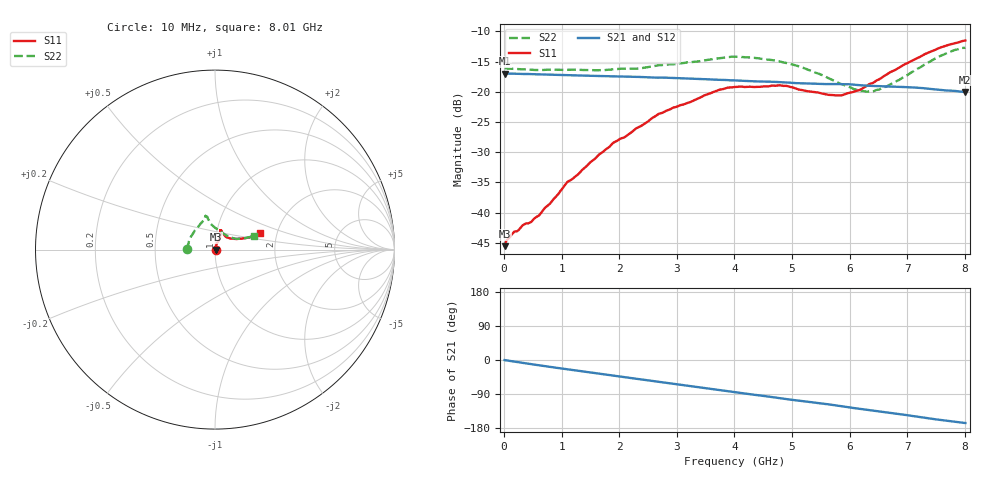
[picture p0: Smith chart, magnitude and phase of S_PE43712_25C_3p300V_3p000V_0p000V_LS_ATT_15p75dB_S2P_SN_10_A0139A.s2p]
! DEVICE ID: PE43712
! File Path: z:\PE43713\PE43713_CHAR_NOM_04292014\AMB\3p300\LS_ATT_15p75dB\PE43713_AMB_3p300V_3p000V_0p000V_LS_ATT_15p75dB_S2P_SN_10_A0139A.s2p
! Serial: 10
! Lot: A0139A
! Temp: 25C
! VDD: 3.300
! VSS: 0.000
! Control_Hi: 3.000
! Control_Lo: 0.000
! Attenuation Step: 15.75dB
! Port 1: RF1
! Port 2: RF2
! ThroughPath:1-2
! IDD: 0.0001475345
! ISS: -1.669e-007
#  Hz  S  RI  R  50
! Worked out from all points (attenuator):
!   801 points, 10 MHz to 8.01 GHz, reference 50 ohm
!   highest |S21| = -16.97 dB at 10 MHz (marker M1); lowest = -20.0 dB at 8 GHz (marker M2)
!   lowest |S11| = -45.6 dB at 10 MHz (marker M3), VSWR 1.01, Z = 50.5 + j0.0439 ohm
!   |S11| at or under -10 dB: start of sweep to end of sweep
!   |S22| runs from -20.0 to -12.7 dB; largest |S21 - S12| = 0.00053
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1e7  0.00525 0.000435  0.1418 -0.000698  0.1419 -0.000719  -0.1568 0.00104
1.6e8  0.00636 0.00237  0.141 -0.00942  0.1411 -0.00942  -0.1547 0.0109
4.6e8  0.00643 0.00528  0.1378 -0.026  0.1378 -0.026  -0.1502 0.0264
6.1e8  0.0059 0.00746  0.1354 -0.0337  0.1354 -0.0338  -0.1475 0.035
9.2e8  0.00499 0.0129  0.1292 -0.0489  0.1293 -0.049  -0.1433 0.0515
1.09e9  0.005 0.017  0.1251 -0.0566  0.1252 -0.0567  -0.1393 0.0612
1.35e9  0.00599 0.0216  0.1184 -0.0677  0.1184 -0.0677  -0.1329 0.0734
1.9e9  0.0116 0.0361  0.1012 -0.0886  0.1011 -0.0886  -0.1141 0.1033
2.34e9  0.0184 0.0476  0.0845 -0.1026  0.0845 -0.1026  -0.0962 0.1232
2.68e9  0.0255 0.0604  0.0705 -0.1105  0.0705 -0.1105  -0.0809 0.1452
3.72e9  0.032 0.0982  0.0238 -0.1236  0.0237 -0.1236  -0.0546 0.1814
4.01e9  0.032 0.105  0.0107 -0.1239  0.0107 -0.1239  -0.0535 0.1879
4.79e9  0.0326 0.1085  -0.0224 -0.1183  -0.0224 -0.1184  -0.0404 0.1738
5.35e9  0.0438 0.0899  -0.0433 -0.1086  -0.0433 -0.1086  -0.0259 0.1461
5.83e9  0.0612 0.0704  -0.0601 -0.0989  -0.0601 -0.099  0.00628 0.117
6.19e9  0.0842 0.0619  -0.0717 -0.0878  -0.0716 -0.0878  0.0401 0.0932
6.4e9  0.1015 0.0608  -0.0765 -0.0816  -0.0764 -0.0816  0.0615 0.0796
6.68e9  0.1299 0.0599  -0.0833 -0.0728  -0.0831 -0.0728  0.0925 0.0659
7.55e9  0.2179 0.0742  -0.0961 -0.0395  -0.0959 -0.0395  0.1834 0.0677
7.81e9  0.2381 0.0829  -0.0972 -0.0305  -0.0972 -0.0305  0.2076 0.0756
8e9  0.2502 0.0892  -0.0967 -0.0238  -0.0966 -0.024  0.2177 0.0781
8.01e9  0.2508 0.0898  -0.0967 -0.0236  -0.0965 -0.0238  0.2183 0.0781
